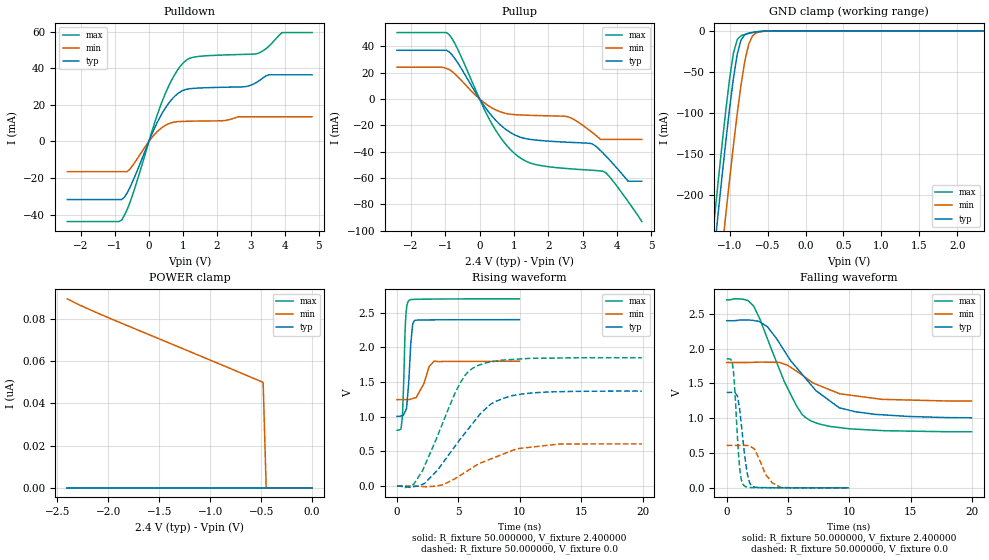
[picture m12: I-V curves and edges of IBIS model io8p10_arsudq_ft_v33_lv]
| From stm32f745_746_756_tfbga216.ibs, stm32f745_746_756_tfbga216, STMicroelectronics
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|   Model io8p10_arsudq_ft_v33_lv
[Model]  io8p10_arsudq_ft_v33_lv
Model_type I/O
Polarity   Non-Inverting
Enable   Active-Low
Vinl =   0.720000V
Vinh =   1.680000V
Vmeas =  1.200000V
Cref =   40.000000pF
Rref =   100.000000M
Vref =   0.0V
C_comp   2.238700pF   2.180600pF   2.332300pF
[Temperature Range]   25.000000   0.125000k   -40.000000
[Pullup Reference]   2.400000V   1.800000V   2.700000V
[Pulldown Reference]   0.0V   0.0V   0.0V
[POWER Clamp Reference]   2.400000V   1.800000V   2.700000V
[GND Clamp Reference]   0.0V   0.0V   0.0V
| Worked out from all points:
|   slope of the pulldown table from 0 to 0.36 V, typ, clamps not added: 25 ohm
|   slope of the pullup table from 0 to 0.36 V, typ, clamps not added: 27.7 ohm
|   GND clamp passes 1 mA (typ) near -0.62 V on its own axis
|   rising waveform, R_fixture 50.000000, V_fixture 2.400000: 20-80 % time 303ps typ, 745ps min, 199ps max; typ from 1.01 V to 2.4 V
|   rising waveform, R_fixture 50.000000, V_fixture 0.0: 20-80 % time 3.62ns typ, 4.16ns min, 2.69ns max; typ from 0 V to 1.37 V
|   falling waveform, R_fixture 50.000000, V_fixture 2.400000: 20-80 % time 3.98ns typ, 3.54ns min, 2.74ns max; typ from 2.4 V to 1.01 V
|   falling waveform, R_fixture 50.000000, V_fixture 0.0: 20-80 % time 534ps typ, 1.04ns min, 387ps max; typ from 1.37 V to 0 V
[Pulldown]
|Voltage   I(typ)   I(min)   I(max)
-2.4V     -31.73mA   -16.51mA   -43.74mA
-800mV    -31.73mA   -16.51mA   -42.87mA
-480mV    -21.98mA   -13.17mA   -29.21mA
80mV      3.63mA     1.966mA    5.014mA
480mV     18.16mA    8.738mA    26.02mA
800mV     25.38mA    10.72mA    37.77mA
1.12V     28.53mA    11.02mA    44.6mA
2.8V      29.84mA    13.47mA    47.53mA
3.2V      32.64mA    13.47mA    48.05mA
3.52V     36.39mA    13.47mA    51.83mA
3.92V     36.39mA    13.47mA    59.44mA
4.8V      36.39mA    13.47mA    59.44mA
[Pullup]
|Voltage   I(typ)   I(min)   I(max)
-2.4V     36.89mA    24.04mA    50.34mA
-960mV    36.89mA    23.04mA    50.34mA
-640mV    27.65mA    17.03mA    38mA
320mV     -11.75mA   -6.207mA   -17.08mA
640mV     -20.52mA   -10.1mA    -30.35mA
960mV     -26.47mA   -11.82mA   -40.02mA
1.52V     -30.88mA   -12.51mA   -49.05mA
2.56V     -32.88mA   -13.48mA   -52.9mA
3.28V     -34.19mA   -25.51mA   -54.18mA
3.6V      -41.31mA   -30.75mA   -54.97mA
4.32V     -62.47mA   -30.75mA   -77.8mA
4.72V     -62.47mA   -30.75mA   -93.1mA
[GND_clamp]
|Voltage   I(typ)   I(min)   I(max)
-2.4V     -1.424A    -1.508A    -1.394A
-1.25V    -311.2mA   -401.9mA   -273.3mA
-1.2V     -265.4mA   -356.1mA   -227.2mA
-1.15V    -220.4mA   -310.8mA   -181.9mA
-1.1V     -176.3mA   -266.2mA   -137.9mA
-1.05V    -133.8mA   -222.5mA   -95.87mA
-950mV    -57.3mA    -138.9mA   -26.98mA
-900mV    -28.27mA   -100.4mA   -10.59mA
-850mV    -11.01mA   -65.54mA   -5.958mA
-750mV    -2.834mA   -16.5mA    -3.178mA
-600mV    -750uA     -1.164mA   -738.3uA
2.35V     0A         0A         0A
[POWER_clamp]
|Voltage   I(typ)   I(min)   I(max)
-2.4V     0A         89.62nA    0A
-2.04V    0A         81.57nA    0A
-480mV    0A         50.01nA    0A
-450mV    0A         0A         0A
0V        0A         0A         0A
[Ramp]
| variable   typ   min   max
dV/dt_r  0.82218/3.62376n   0.36588/4.16745n   1.11108/2.68940n
dV/dt_f  0.83424/3.99209n   0.33390/3.59548n   1.13659/2.74073n
R_load = 50.000000
[Rising Waveform]
R_fixture= 50.000000
V_fixture= 2.400000
V_fixture_min= 1.800000
V_fixture_max= 2.700000
|time   V(typ)   V(min)   V(max)
0s        1.006V     1.247V     804.9mV
320.3ps   1.01V      1.247V     822.9mV
440.4ps   1.016V     1.247V     1.002V
680.7ps   1.081V     1.247V     2.333V
800.8ps   1.172V     1.246V     2.599V
961ps     1.514V     1.246V     2.674V
1.121ns   2.055V     1.255V     2.689V
1.421ns   2.387V     1.27V      2.693V
3.023ns   2.397V     1.801V     2.697V
9.97ns    2.4V       1.8V       2.7V
[Rising Waveform]
R_fixture= 50.000000
V_fixture= 0.0
V_fixture_min= 0.0
V_fixture_max= 0.0
|time   V(typ)   V(min)   V(max)
0s        74.64uV    35.05uV    234.7uV
1.361ns   -7.745mV   -507.2uV   28.06mV
2.042ns   23.59mV    -6.465mV   210.8mV
3.283ns   227.4mV    3.25mV     716.4mV
4.805ns   595.7mV    116mV      1.371V
5.566ns   770.6mV    201mV      1.602V
6.326ns   940.4mV    286mV      1.716V
7.608ns   1.179V     389.3mV    1.789V
9.77ns    1.317V     538.9mV    1.83V
19.94ns   1.37V      609.1mV    1.851V
[Falling Waveform]
R_fixture= 50.000000
V_fixture= 2.400000
V_fixture_min= 1.800000
V_fixture_max= 2.700000
|time   V(typ)   V(min)   V(max)
0s        2.4V       1.8V       2.7V
1.642ns   2.41V      1.8V       2.694V
2.202ns   2.403V     1.802V     2.607V
3.323ns   2.311V     1.805V     2.137V
4.725ns   1.958V     1.775V     1.512V
6.126ns   1.634V     1.621V     1.058V
6.767ns   1.5V       1.54V      970.6mV
9.169ns   1.149V     1.353V     865.3mV
10.45ns   1.094V     1.322V     843.1mV
19.94ns   1.006V     1.247V     804.9mV
[Falling Waveform]
R_fixture= 50.000000
V_fixture= 0.0
V_fixture_min= 0.0
V_fixture_max= 0.0
|time   V(typ)   V(min)   V(max)
0s        1.37V      609.1mV    1.851V
460.5ps   1.371V     609mV      1.79V
660.7ps   1.366V     608.9mV    1.397V
1.041ns   1.145V     608.6mV    313.1mV
1.421ns   521.7mV    609.5mV    31.04mV
1.802ns   107.2mV    605.6mV    7.042mV
2.202ns   14.73mV    563.4mV    3.641mV
3.143ns   2.485mV    198.9mV    1.947mV
4.364ns   1.207mV    9.873mV    1.11mV
9.97ns    74.64uV    35.05uV    234.7uV
